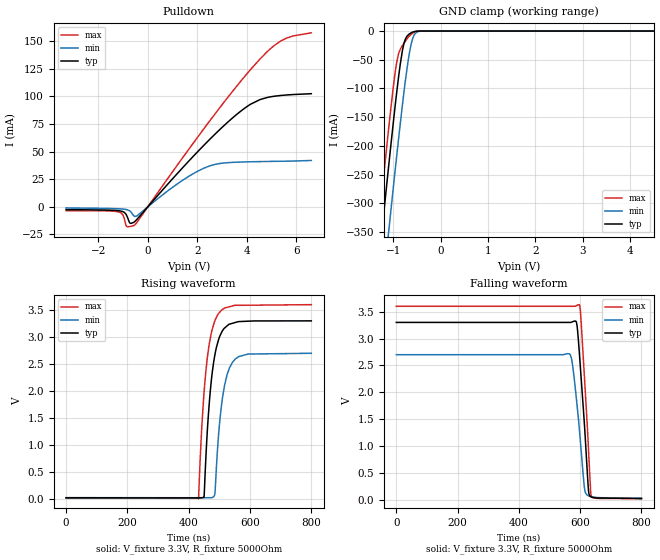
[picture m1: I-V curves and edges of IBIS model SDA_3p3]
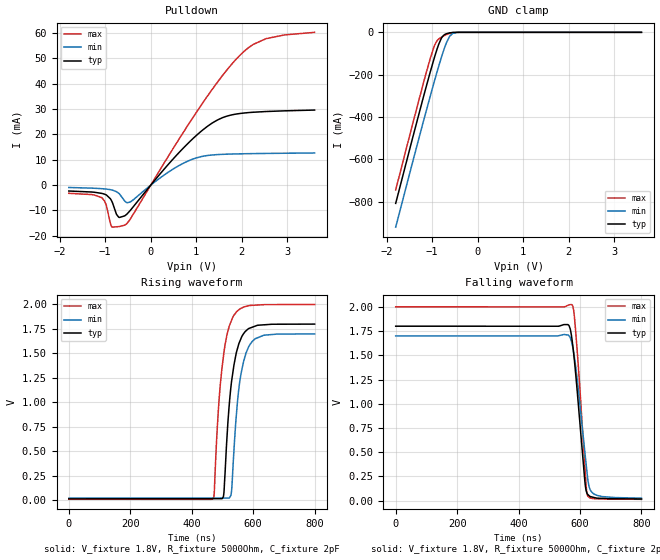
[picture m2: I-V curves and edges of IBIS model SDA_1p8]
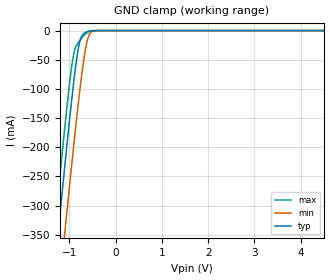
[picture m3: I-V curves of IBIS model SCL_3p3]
[IBIS Ver]   4.1
[File name]   tmp451q1.ibs
[File Rev]   1.0
[Date]   08/02/2024
[Source]
| Texas Instruments Incorporated.
| 12500 TI Blvd
| Dallas, TX -75243
[Notes]   Revision History:
| Rev 1.0: 08/01/2024
| - Initial version of the model
| - Model generated from simulations in TISPICE
| - C_comp although listed in numerical order of value are
|   obtained from varying PVT conditions. For PVT conditions for
|   each specific value refer the buffer description under
|   respective [Model]. IBIS model user is responsible for using
|   appropriate C_comp to simulate for Signal Integrity.
| - Warnings regarding combined Non-monotonicity of various models have been
|   reviewd and considered minor and can be ignored.
| -  Model names with a trailing _3p3 contains the model
|   for 3.3V operation. Model names with a trailing _5p5 contains the model
|   for 5.5V operation.
[Disclaimer]
| This model is designed as an aid for customers of Texas Instruments.
| TI and its licensors and suppliers make no warranties, either expressed
| or implied, with respect to this  model, including the warranties of
| merchantability or fitness for a particular purpose. The model is
| provided solely on an "as is" basis. The entire risk as to its quality
| and performance is with the customer.
[Copyright]
 (C) Copyright 2024 Texas Instruments Incorporated.All rights reserved.
|   Device
[Component]   TMP451Q-1
[Manufacturer]   TI
[Package]   |DQW 8 pin
| variable   typ   min   max
R_pkg   0.083   0.076   0.088
L_pkg   1.774nH   1.670nH   1.869nH
C_pkg   0.393pF   0.385pF   0.402pF
[Pin]  signal_name   model_name   R_pin   L_pin   C_pin
1   SDA   SDA   0.08836   1.8688nH   0.38537pF
2   SCL   SCL   0.0798   1.72452nH   0.40219pF
3   ALERT   ALERT   0.07626   1.67019nH   0.40077pF
4   T_CRIT   T_CRIT   0.07626   1.67019nH   0.40077pF
5   GND   GND   0.08804   1.86388nH   0.38801pF
6   V+   POWER   0.08723   1.84409nH   0.38521pF
|   Model Selectors
[Model Selector]  SDA
SDA_3p3  SDA buffer at 5.5V operation.
SDA_1p8  SDA buffer at 3.3V operation.
[Model Selector]  SCL
SCL_3p3  SCL buffer at 5.5V operation.
SCL_1p8  SCL buffer at 3.3V operation.
[Model Selector]  T_CRIT
T_CRIT_3p3  TCRIT buffer at 5.5V operation.
T_CRIT_1p8  TCRIT buffer at 3.3V operation.
[Model Selector]  ALERT
ALERT_3p3  ALERT buffer at 5.5V operation.
ALERT_1p8  ALERT buffer at 3.3V operation.
| Models and submodels in the file (8): SDA_3p3 (I/O_open_drain), SDA_1p8 (I/O_open_drain), SCL_3p3 (Input), SCL_1p8 (Input), T_CRIT_3p3 (Open_drain), T_CRIT_1p8 (Open_drain), ALERT_3p3 (Open_drain), ALERT_1p8 (Open_drain)
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|   Model
[Model]   SDA_3p3
Model_type   I/O_open_drain
Polarity   Non-Inverting
Enable   Active-Low
Vinl = .45
Vinh = 1.4
Vmeas = 1.65
Vref = 3.30
Cref = 2pF
Rref = 5000
|   typ   min   max
C_comp   1.69pF   1.64pF   1.76pF
[Voltage Range]   3.3   2.7   3.6
[Temperature Range]   25   125   -40
[Pullup Reference]   3.3   2.7   3.6
[Pulldown Reference]   0   -0   0
[Power Clamp Reference]   3.3   2.7   3.6
[GND Clamp Reference]   0   0   0
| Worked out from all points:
|   slope of the pulldown table from 0 to 0.495 V, typ, clamps not added: 39 ohm
|   GND clamp passes 1 mA (typ) near -0.56 V on its own axis
|   falling waveform, V_fixture 3.3V, R_fixture 5000Ohm: 20-80 % time 23.1ns typ, 26ns min, 21.3ns max; typ from 3.3 V to 0.026 V
|   rising waveform, V_fixture 3.3V, R_fixture 5000Ohm: 20-80 % time 29.3ns typ, 29.2ns min, 30.1ns max; typ from 0.025 V to 3.3 V
[Pulldown]
|   Voltage   I(typ)   I(min)   I(max)
-3.3V     -2.52mA    -1.007mA   -3.483mA
-1.171V   -3.568mA   -1.79mA    -4.632mA
-1.003V   -4.391mA   -2.058mA   -7.469mA
-874.5mV  -6.884mA   -2.452mA   -17.4mA
-716.1mV  -14.76mA   -3.957mA   -17.8mA
-537.9mV  -13.54mA   -8.544mA   -16.53mA
2.095V    51.82mA    33.15mA    65.61mA
2.788V    67.42mA    38.75mA    86.3mA
3.897V    89.05mA    40.62mA    117.6mA
4.531V    97.07mA    40.94mA    133.8mA
5.343V    100.7mA    41.22mA    149.8mA
6.6V      102.4mA    41.95mA    157.5mA
[GND Clamp]
|   Voltage   I(typ)   I(min)   I(max)
-3.3V     -2.079A    -2.184A    -2.023A
-1.379V   -459.2mA   -573.9mA   -393.5mA
-1.211V   -322.2mA   -437.2mA   -256.2mA
-1.102V   -235.5mA   -350.1mA   -170.1mA
-943.8mV  -115.3mA   -226.6mA   -60.78mA
-884.4mV  -74.88mA   -181.9mA   -37.49mA
-815.1mV  -36.05mA   -131.6mA   -25.91mA
-735.9mV  -12.09mA   -78.72mA   -16.07mA
-607.2mV  -2.337mA   -16.65mA   -4.359mA
-528mV    -485.7uA   -3.278mA   -849.8uA
-399.3mV  -8.979uA   -124.6uA   -5.992uA
6.6V      0A         0A         0A
[Ramp]
R_load = 5000
|   typ   min   max
dV/dt_r   1.96477/2.93375e-08   1.60285/2.90224e-08   2.1466/2.99953e-08
dV/dt_f   1.96443/2.30555e-08   1.60196/2.59999e-08   2.14647/2.12879e-08
[Falling Waveform]
V_fixture = 3.3V
V_fixture_min = 2.7V
V_fixture_max = 3.6V
R_fixture = 5000Ohm
C_fixture = 0F
|   Time   V(typ)   V(min)   V(max)
0s        3.3V       2.7V       3.6V
564.8ns   3.3V       2.716V     3.6V
574.6ns   3.311V     2.531V     3.6V
587.5ns   3.306V     1.891V     3.611V
597ns     2.752V     1.331V     3.63V
601.1ns   2.429V     1.06V      3.484V
615.2ns   1.281V     180mV      2.153V
627.1ns   180.7mV    75.66mV    949.5mV
636.2ns   54.03mV    61.38mV    70.39mV
800ns     25.94mV    30.06mV    22.55mV
[Rising Waveform]
V_fixture = 3.3V
V_fixture_min = 2.7V
V_fixture_max = 3.6V
R_fixture = 5000Ohm
C_fixture = 0F
|   Time   V(typ)   V(min)   V(max)
0s        25.3mV     28.48mV    22.28mV
432.1ns   22.95mV    26.33mV    9.025mV
450ns     34.3mV     26.24mV    1.969V
457.4ns   926mV      26.21mV    2.447V
470.5ns   2.003V     26.14mV    2.973V
485.5ns   2.674V     99.21mV    3.304V
494.7ns   2.897V     977.6mV    3.412V
517.2ns   3.168V     2.113V     3.537V
552ns     3.27V      2.594V     3.587V
800ns     3.3V       2.7V       3.6V
|   Model
[Model]   SDA_1p8
Model_type   I/O_open_drain
Polarity   Non-Inverting
Enable   Active-Low
Vinl = .45
Vinh = 1.4
Vmeas = 0.9
Vref = 1.8
Cref = 2pF
Rref = 5000
|   typ   min   max
C_comp   1.91pF   1.78pF   2.04pF
[Voltage Range]   1.8   1.7   2
[Temperature Range]   25   125   -40
[Pullup Reference]   1.8   1.7   2
[Pulldown Reference]   0   0   0
[Power Clamp Reference]   1.8   1.7   2
[GND Clamp Reference]   0   0   0
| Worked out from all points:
|   slope of the pulldown table from 0 to 0.27 V, typ, clamps not added: 46.5 ohm
|   GND clamp passes 1 mA (typ) near -0.56 V on its own axis
|   falling waveform, V_fixture 1.8V, R_fixture 5000Ohm, C_fixture 2pF: 20-80 % time 29.3ns typ, 33.8ns min, 25.2ns max; typ from 1.8 V to 0.017 V
|   rising waveform, V_fixture 1.8V, R_fixture 5000Ohm, C_fixture 2pF: 20-80 % time 31.1ns typ, 30.6ns min, 31.5ns max; typ from 0.016 V to 1.8 V
[Pulldown]
|   Voltage   I(typ)   I(min)   I(max)
-1.8V     -2.313mA   -922.5uA   -3.215mA
-1.076V   -3.247mA   -1.39mA    -4.928mA
-979.2mV  -3.826mA   -1.548mA   -7.765mA
-855mV    -6.368mA   -1.89mA    -16.4mA
-703.8mV  -12.65mA   -3.181mA   -16.35mA
-541.8mV  -11.71mA   -6.743mA   -15.43mA
462.6mV   9.753mA    6.026mA    13.63mA
991.8mV   19.45mA    10.7mA     28.45mA
1.445V    25.52mA    12.04mA    40.15mA
1.948V    28.26mA    12.36mA    51.06mA
2.531V    29.07mA    12.52mA    57.81mA
3.6V      29.64mA    12.7mA     60.33mA
[GND Clamp]
|   Voltage   I(typ)   I(min)   I(max)
-1.8V     -808.9mA   -921.3mA   -745.2mA
-1.201V   -313.8mA   -428.8mA   -247.8mA
-1.044V   -190.2mA   -304.2mA   -126.2mA
-973.8mV  -137.1mA   -249.6mA   -78.08mA
-936mV    -109.8mA   -220.7mA   -56.8mA
-887.4mV  -76.81mA   -184.1mA   -38.27mA
-779.4mV  -22.17mA   -107mA     -21.32mA
-687.6mV  -6.678mA   -50.63mA   -10.95mA
-617.4mV  -2.726mA   -19.81mA   -5.043mA
-547.2mV  -762.6uA   -5.034mA   -1.396mA
-363.6mV  -2.439uA   -45.93uA   -1.107uA
3.6V      0A         0A         0A
[Ramp]
R_load = 5000
|   typ   min   max
dV/dt_r   1.07021/3.08893e-08   1.00591/3.04457e-08   1.19201/3.14737e-08
dV/dt_f   1.06975/2.92594e-08   1.00441/3.37531e-08   1.19187/2.51697e-08
[Falling Waveform]
V_fixture = 1.8V
V_fixture_min = 1.7V
V_fixture_max = 2V
R_fixture = 5000Ohm
C_fixture = 2pF
|   Time   V(typ)   V(min)   V(max)
0s        1.8V       1.7V       2V
560.6ns   1.817V     1.709V     2.015V
574.2ns   1.656V     1.614V     2.02V
579.4ns   1.516V     1.527V     1.962V
586.4ns   1.291V     1.372V     1.727V
615.7ns   200.4mV    501.6mV    352.5mV
624.5ns   66.81mV    241.6mV    53.12mV
634.4ns   41.52mV    105.1mV    25.92mV
656.2ns   25.69mV    53.36mV    18.22mV
800ns     17.08mV    25.98mV    13.55mV
[Rising Waveform]
V_fixture = 1.8V
V_fixture_min = 1.7V
V_fixture_max = 2V
R_fixture = 5000Ohm
C_fixture = 2pF
|   Time   V(typ)   V(min)   V(max)
0s        16.23mV    23.36mV    13.25mV
469.8ns   18.95mV    23.95mV    18.16mV
473.4ns   18.97mV    23.95mV    78.11mV
488.6ns   19.06mV    23.97mV    1.007V
503.2ns   38.87mV    23.99mV    1.469V
527.2ns   1.144V     48.99mV    1.819V
533.6ns   1.298V     296.2mV    1.87V
555.9ns   1.618V     1.2V       1.953V
589.1ns   1.759V     1.589V     1.99V
800ns     1.8V       1.7V       2V
|   Model
[Model]   SCL_3p3
Model_type   Input
Vinl = .45
Vinh = 1.4
|   typ   min   max
C_comp   1.34pF   1.32pF   1.35pF
[Voltage Range]   3.3   2.7   3.6
[Temperature Range]   25   125   -40
[Power Clamp Reference]   3.3   2.7   3.6
[GND Clamp Reference]   0   0   0
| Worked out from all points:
|   GND clamp passes 1 mA (typ) near -0.58 V on its own axis
[GND Clamp]
|   Voltage   I(typ)   I(min)   I(max)
-3.3V     -2.077A    -2.182A    -2.02A
-1.379V   -458.1mA   -572.6mA   -391.8mA
-1.211V   -321.1mA   -436mA     -254.4mA
-1.102V   -234.4mA   -349mA     -168.2mA
-1.092V   -226.6mA   -341.1mA   -160.6mA
-993.3mV  -150.5mA   -263.6mA   -88mA
-894.3mV  -79.88mA   -188.2mA   -35.59mA
-775.5mV  -18.9mA    -103.2mA   -17.04mA
-627mV    -2.193mA   -21.72mA   -4.275mA
-547.8mV  -486.9uA   -4.124mA   -939uA
-419.1mV  -10.31uA   -127.6uA   -8.322uA
6.6V      0A         0A         0A
